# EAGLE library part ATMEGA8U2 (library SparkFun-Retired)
Atmel 32-pin 8-bit Microcontroller with 8/16/32K Bystes of ISP Flash and USB Controller. ATmega8U2, ATmega16U2, and ATmega32U2 Datasheet SparkFun Products Storefront component: ATMEGA8U2-AU (COM-13703)
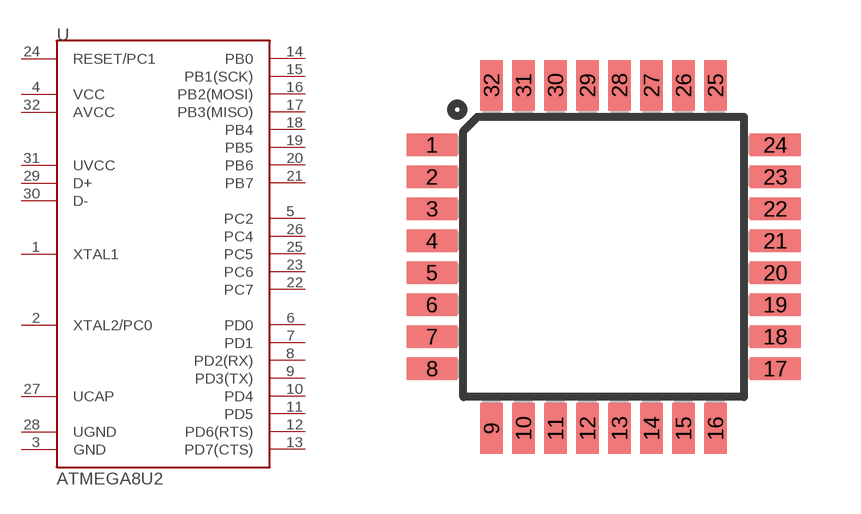
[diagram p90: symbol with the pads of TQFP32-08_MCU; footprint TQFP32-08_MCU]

Designator prefix U

## ATMEGA8U2AU (PROD_ID: IC-10104; VALUE: 8U2-AU)  [TQFP32-08_MCU]
1  XTAL1
2  XTAL2/PC0
3  GND
4  VCC
5  PC2
6  PD0
7  PD1
8  PD2(RX)
9  PD3(TX)
10  PD4
11  PD5
12  PD6(RTS)
13  PD7(CTS)
14  PB0
15  PB1(SCK)
16  PB2(MOSI)
17  PB3(MISO)
18  PB4
19  PB5
20  PB6
21  PB7
22  PC7
23  PC6
24  RESET/PC1
25  PC5
26  PC4
27  UCAP
28  UGND
29  D+
30  D-
31  UVCC
32  AVCC

## Footprint TQFP32-08_MCU (pad centres in mm)
Thin Plasic Quad Flat Package Grid 0.8 mm
smd 1.27 x 0.559: 1 -4.293,2.8; 2 -4.293,2; 3 -4.293,1.2; 4 -4.293,0.4; 5 -4.293,-0.4; 6 -4.293,-1.2; 7 -4.293,-2; 8 -4.293,-2.8; 17 4.293,-2.8; 18 4.293,-2; 19 4.293,-1.2; 20 4.293,-0.4; 21 4.293,0.4; 22 4.293,1.2; 23 4.293,2; 24 4.293,2.8
smd 0.559 x 1.27: 9 -2.8,-4.293; 10 -2,-4.293; 11 -1.2,-4.293; 12 -0.4,-4.293; 13 0.4,-4.293; 14 1.2,-4.293; 15 2,-4.293; 16 2.8,-4.293; 25 2.8,4.293; 26 2,4.293; 27 1.2,4.293; 28 0.4,4.293; 29 -0.4,4.293; 30 -1.2,4.293; 31 -2,4.293; 32 -2.8,4.293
